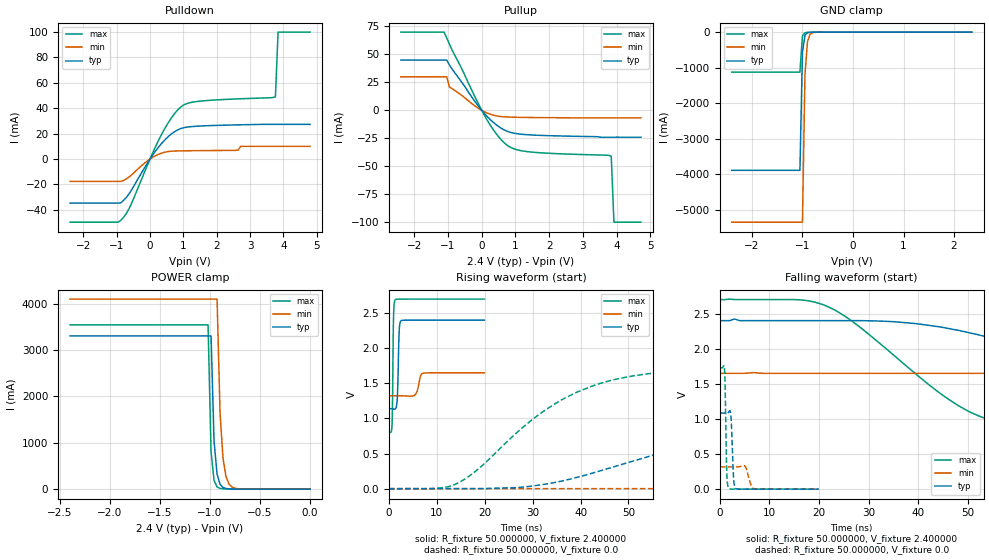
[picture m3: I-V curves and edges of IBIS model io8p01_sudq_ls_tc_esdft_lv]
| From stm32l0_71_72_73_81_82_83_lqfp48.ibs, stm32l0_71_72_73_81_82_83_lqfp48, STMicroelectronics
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|   Model io8p01_sudq_ls_tc_esdft_lv
[Model]  io8p01_sudq_ls_tc_esdft_lv
Model_type I/O
Polarity   Non-Inverting
Enable   Active-Low
Vinl =   0.720000V
Vinh =   1.680000V
Vmeas =  1.200000V
Cref =   50.000000pF
Rref =   100.000000M
Vref =   0.0V
C_comp   2.242700pF   2.201100pF   2.288600pF
[Temperature Range]   25.000000   0.105000k   -40.000000
[Pullup Reference]   2.400000V   1.650000V   2.700000V
[Pulldown Reference]   0.0V   0.0V   0.0V
[POWER Clamp Reference]   2.400000V   1.650000V   2.700000V
[GND Clamp Reference]   0.0V   0.0V   0.0V
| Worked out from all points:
|   slope of the pulldown table from 0 to 0.36 V, typ, clamps not added: 28.4 ohm
|   slope of the pullup table from 0 to 0.36 V, typ, clamps not added: 32.2 ohm
|   GND clamp passes 1 mA (typ) near -0.65 V on its own axis
|   POWER clamp passes 1 mA (typ) near -0.63 V on its own axis
|   rising waveform, R_fixture 50.000000, V_fixture 2.400000: 20-80 % time 279ps typ, 629ps min, 186ps max; typ from 1.14 V to 2.4 V
|   rising waveform, R_fixture 50.000000, V_fixture 0.0: 20-80 % time 40.5ns typ, 109ns min, 19.8ns max; typ from 0 V to 1.08 V
|   falling waveform, R_fixture 50.000000, V_fixture 2.400000: 20-80 % time 41.1ns typ, 105ns min, 20.2ns max; typ from 2.4 V to 1.14 V
|   falling waveform, R_fixture 50.000000, V_fixture 0.0: 20-80 % time 354ps typ, 756ps min, 262ps max; typ from 1.08 V to 0 V
[Pulldown]
|Voltage   I(typ)   I(min)   I(max)
-2.4V     -34.7mA    -17.62mA   -49.77mA
-880mV    -34.55mA   -17.62mA   -48.41mA
-560mV    -24.66mA   -12.69mA   -35.31mA
240mV     8.893mA    3.542mA    13.9mA
560mV     17.98mA    5.931mA    29.16mA
880mV     23.57mA    6.389mA    40.03mA
1.44V     25.89mA    6.593mA    45.41mA
2.64V     26.92mA    7mA        47.38mA
2.72V     26.96mA    10mA       47.46mA
3.76V     27.3mA     10mA       49mA
3.84V     27.3mA     10mA       100mA
4.8V      27.3mA     10mA       100mA
[Pullup]
|Voltage   I(typ)   I(min)   I(max)
-2.4V     45mA       30mA       70mA
-1.12V    45mA       30mA       70mA
-1.04V    45mA       30mA       64.8mA
-960mV    40.7mA     21mA       59.3mA
80mV      -2.838mA   -1.261mA   -4.478mA
480mV     -14.04mA   -5.167mA   -22.91mA
800mV     -19.2mA    -5.978mA   -32.18mA
1.04V     -20.85mA   -6.184mA   -35.23mA
1.44V     -21.93mA   -6.373mA   -37.19mA
3.84V     -24mA      -6.7mA     -41mA
3.92V     -24mA      -6.7mA     -100mA
4.72V     -24mA      -6.7mA     -100mA
[GND_clamp]
|Voltage   I(typ)   I(min)   I(max)
-2.4V     -3.892A    -5.353A    -1.127A
-1.05V    -3.892A    -5.353A    -1.127A
-1V       -568.8mA   -5.353A    -105.4mA
-950mV    -88.95mA   -1.19A     -18.03mA
-900mV    -18.15mA   -269.2mA   -8.959mA
-850mV    -6.699mA   -63.45mA   -6.568mA
-800mV    -4.014mA   -16.61mA   -4.858mA
-650mV    -1.043mA   -1.218mA   -1.146mA
2.35V     0A         0A         0A
[POWER_clamp]
|Voltage   I(typ)   I(min)   I(max)
-2.4V     3.303A     4.097A     3.542A
-1.02V    3.303A     4.097A     3.542A
-990mV    3.303A     4.097A     802.4mA
-960mV    1.032A     4.097A     186.5mA
-930mV    325.2mA    4.097A     47.59mA
-900mV    104.8mA    1.637A     15.78mA
-870mV    35.83mA    655.7mA    8.015mA
-840mV    13.93mA    263.9mA    5.668mA
-810mV    6.712mA    107.2mA    4.56mA
-780mV    4.088mA    44.39mA    3.763mA
-690mV    1.741mA    4.361mA    1.91mA
0V        0A         0A         0A
[Ramp]
| variable   typ   min   max
dV/dt_r  0.65070/40.49041n   0.18965/0.10898u   1.03800/19.79849n
dV/dt_f  0.75696/41.02482n   0.19470/0.10539u   1.13786/20.21446n
R_load = 50.000000
[Rising Waveform]
R_fixture= 50.000000
V_fixture= 2.400000
V_fixture_min= 1.650000
V_fixture_max= 2.700000
|time   V(typ)   V(min)   V(max)
0s        1.139V     1.322V     803.4mV
680.7ps   1.138V     1.322V     928.8mV
961ps     1.134V     1.322V     2.397V
1.321ns   1.133V     1.322V     2.689V
1.762ns   1.294V     1.322V     2.698V
2.162ns   2.249V     1.322V     2.699V
2.523ns   2.39V      1.322V     2.699V
5.526ns   2.4V       1.341V     2.7V
7.167ns   2.4V       1.643V     2.7V
19.94ns   2.4V       1.65V      2.7V
[Rising Waveform]
R_fixture= 50.000000
V_fixture= 0.0
V_fixture_min= 0.0
V_fixture_max= 0.0
|time   V(typ)   V(min)   V(max)
0s        14.03uV    -3.523uV   -8.582uV
14.01ns   -165.2uV   -35.76uV   66.59mV
32.03ns   56.87mV    -35.13uV   1.091V
43.04ns   232.3mV    -34.56uV   1.476V
54.05ns   454.6mV    -29.23uV   1.636V
66.07ns   666.4mV    104.9uV    1.698V
94.09ns   950.8mV    1.595mV    1.728V
138.1ns   1.068V     48.45mV    1.73V
276.3ns   1.085V     273.5mV    1.73V
498.5ns   1.085V     316.6mV    1.73V
[Falling Waveform]
R_fixture= 50.000000
V_fixture= 2.400000
V_fixture_min= 1.650000
V_fixture_max= 2.700000
|time   V(typ)   V(min)   V(max)
0s        2.4V       1.65V      2.7V
21.02ns   2.4V       1.65V      2.622V
35.04ns   2.385V     1.65V      1.909V
50.05ns   2.231V     1.65V      1.11V
57.06ns   2.109V     1.65V      945.9mV
67.07ns   1.905V     1.65V      870.3mV
96.1ns    1.39V      1.65V      817mV
137.1ns   1.199V     1.636V     805.2mV
281.3ns   1.139V     1.388V     803.4mV
498.5ns   1.139V     1.322V     803.4mV
[Falling Waveform]
R_fixture= 50.000000
V_fixture= 0.0
V_fixture_min= 0.0
V_fixture_max= 0.0
|time   V(typ)   V(min)   V(max)
0s        1.085V     316.6mV    1.73V
961ps     1.085V     316.6mV    1.722V
1.121ns   1.084V     316.6mV    1.371V
1.401ns   1.084V     316.6mV    287.9mV
1.802ns   1.097V     316.6mV    14.53mV
2.242ns   1.056V     316.6mV    1.297mV
2.803ns   152.5mV    316.4mV    553.3uV
3.243ns   8.571mV    316mV      421.4uV
6.887ns   58.76uV    5.899mV    17uV
19.94ns   14.03uV    -3.523uV   -8.582uV
